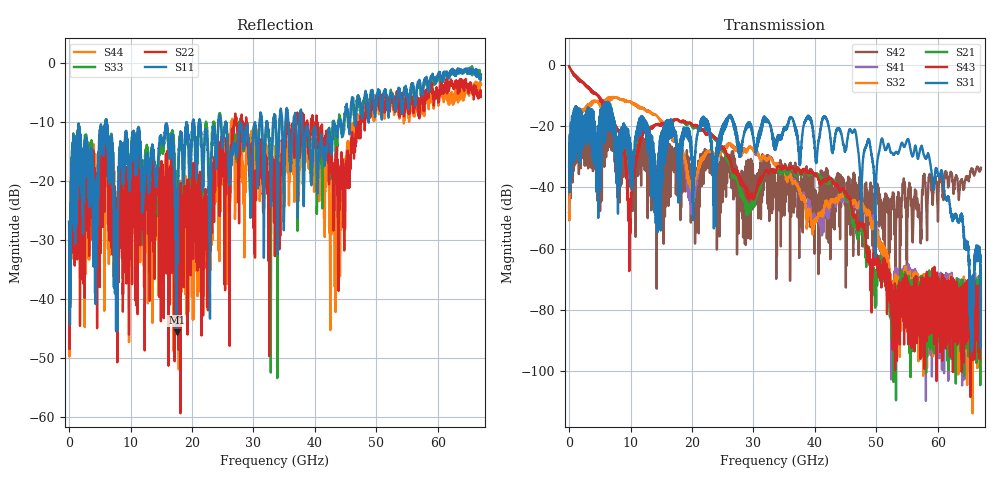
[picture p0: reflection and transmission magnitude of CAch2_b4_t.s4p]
!Agilent Technologies,N5247A,US51170199,A.09.90.13
!Agilent N5247A: A.09.90.13
!Date: Tuesday, October 23, 2018 13:18:06
!Correction: S11(Full 4 Port(1,2,3,4))
!S12(Full 4 Port(1,2,3,4))
!S13(Full 4 Port(1,2,3,4))
!S14(Full 4 Port(1,2,3,4))
!S21(Full 4 Port(1,2,3,4))
!S22(Full 4 Port(1,2,3,4))
!S23(Full 4 Port(1,2,3,4))
!S24(Full 4 Port(1,2,3,4))
!S31(Full 4 Port(1,2,3,4))
!S32(Full 4 Port(1,2,3,4))
!S33(Full 4 Port(1,2,3,4))
!S34(Full 4 Port(1,2,3,4))
!S41(Full 4 Port(1,2,3,4))
!S42(Full 4 Port(1,2,3,4))
!S43(Full 4 Port(1,2,3,4))
!S44(Full 4 Port(1,2,3,4))
!S4P File: Measurements: <S11,S12,S13,S14>,
!<S21,S22,S23,S24>,
!<S31,S32,S33,S34>,
!<S41,S42,S43,S44>:
# Hz S  dB  R 50
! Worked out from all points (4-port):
!   6701 points, 10 MHz to 67 GHz, reference 50 ohm
!   strongest paths, dB at 10 MHz, 16.76 GHz, 33.51 GHz, 50.25 GHz, 67 GHz:
!     S31: -33.1, -22.6, -25.7, -30.2, -68.1
!     S43: -0.4, -18.2, -35.1, -62.5, -79.1
!     S21: -0.4, -18.0, -35.2, -64.0, -77.2
!     S32: -48.3, -23.6, -32.7, -55.0, -81.1
!     S41: -48.4, -23.9, -32.9, -54.5, -79.1
!     S42: -33.5, -34.0, -38.2, -45.3, -33.6
!   lowest |S11| = -45.7 dB at 17.51 GHz (marker M1), VSWR 1.01, Z = 50.3 + j0.426 ohm
!   |S11| at or under -10 dB: start of sweep to 5.978 GHz; 6.104 GHz to 20.15 GHz (14.05 GHz wide, 107 % of centre); 24.69 GHz to 31.02 GHz (6.331 GHz wide, 22.7 % of centre)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
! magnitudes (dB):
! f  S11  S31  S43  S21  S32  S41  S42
! 10 MHz  -26.9  -33.1  -0.4  -0.4  -48.3  -48.4  -33.5
! 1.89 GHz  -16.7  -31.8  -5.1  -5.1  -15.9  -15.9  -33.8
! 9.839 GHz  -19.2  -30.1  -48.2  -33.0  -12.0  -11.9  -31.2
! 17.51 GHz  -45.7  -24.7  -17.9  -17.8  -25.4  -25.6  -32.7
! 42.55 GHz  -14.6  -24.0  -37.0  -37.8  -45.1  -45.3  -43.6
! 55.1 GHz  -6.0  -24.3  -85.1  -70.7  -74.6  -77.0  -49.0
! 67 GHz  -2.0  -68.1  -79.1  -77.2  -81.1  -79.1  -33.6
